DATA_BLOCK "BreukData"
TITLE =
VERSION : 0.1


  STRUCT
   Leiding : ARRAY  [0 .. 100 ] OF //Drukwaarde
   REAL  := 0.000000e+000;
  END_STRUCT ;
BEGIN
Leiding[0] := 	0.14354;
Leiding[1] := 	0.14587;
Leiding[2] := 	0.14940;
Leiding[3] := 	0.15412;
Leiding[4] := 	0.16004;
Leiding[5] := 	0.16715;
Leiding[6] := 	0.17545;
Leiding[7] := 	0.18494;
Leiding[8] := 	0.19563;
Leiding[9] := 	0.20752;
Leiding[10] := 	0.22059;
Leiding[11] := 	0.23487;
Leiding[12] := 	0.25033;
Leiding[13] := 	0.26699;
Leiding[14] := 	0.28484;
Leiding[15] := 	0.30389;
Leiding[16] := 	0.32413;
Leiding[17] := 	0.34556;
Leiding[18] := 	0.36819;
Leiding[19] := 	0.39201;
Leiding[20] := 	0.41702;
Leiding[21] := 	0.44323;
Leiding[22] := 	0.47063;
Leiding[23] := 	0.49923;
Leiding[24] := 	0.52902;
Leiding[25] := 	0.56000;
Leiding[26] := 	0.59218;
Leiding[27] := 	0.62555;
Leiding[28] := 	0.66011;
Leiding[29] := 	0.69587;
Leiding[30] := 	0.73282;
Leiding[31] := 	0.77097;
Leiding[32] := 	0.81031;
Leiding[33] := 	0.85084;
Leiding[34] := 	0.89257;
Leiding[35] := 	0.93549;
Leiding[36] := 	0.97960;
Leiding[37] := 	1.02491;
Leiding[38] := 	1.07141;
Leiding[39] := 	1.11911;
Leiding[40] := 	1.16800;
Leiding[41] := 	1.21808;
Leiding[42] := 	1.26936;
Leiding[43] := 	1.32183;
Leiding[44] := 	1.37549;
Leiding[45] := 	1.43035;
Leiding[46] := 	1.48640;
Leiding[47] := 	1.54364;
Leiding[48] := 	1.60208;
Leiding[49] := 	1.66172;
Leiding[50] := 	1.72254;
Leiding[51] := 	1.78456;
Leiding[52] := 	1.84778;
Leiding[53] := 	1.91218;
Leiding[54] := 	1.97778;
Leiding[55] := 	2.04458;
Leiding[56] := 	2.11257;
Leiding[57] := 	2.18175;
Leiding[58] := 	2.25213;
Leiding[59] := 	2.32370;
Leiding[60] := 	2.39646;
Leiding[61] := 	2.47042;
Leiding[62] := 	2.54557;
Leiding[63] := 	2.62191;
Leiding[64] := 	2.69945;
Leiding[65] := 	2.77818;
Leiding[66] := 	2.85811;
Leiding[67] := 	2.93923;
Leiding[68] := 	3.02154;
Leiding[69] := 	3.10505;
Leiding[70] := 	3.18975;
Leiding[71] := 	3.27565;
Leiding[72] := 	3.36274;
Leiding[73] := 	3.45102;
Leiding[74] := 	3.54049;
Leiding[75] := 	3.63116;
Leiding[76] := 	3.72303;
Leiding[77] := 	3.81608;
Leiding[78] := 	3.91033;
Leiding[79] := 	4.00578;
Leiding[80] := 	4.10242;
Leiding[81] := 	4.20025;
Leiding[82] := 	4.29927;
Leiding[83] := 	4.39949;
Leiding[84] := 	4.50091;
Leiding[85] := 	4.60351;
Leiding[86] := 	4.70731;
Leiding[87] := 	4.81231;
Leiding[88] := 	4.91850;
Leiding[89] := 	5.02588;
Leiding[90] := 	5.13445;
Leiding[91] := 	5.24422;
Leiding[92] := 	5.35519;
Leiding[93] := 	5.46734;
Leiding[94] := 	5.58069;
Leiding[95] := 	5.69524;
Leiding[96] := 	5.81098;
Leiding[97] := 	5.92791;
Leiding[98] := 	6.04603;
Leiding[99] := 	6.16535;
Leiding[100] := 6.28586;
END_DATA_BLOCK

